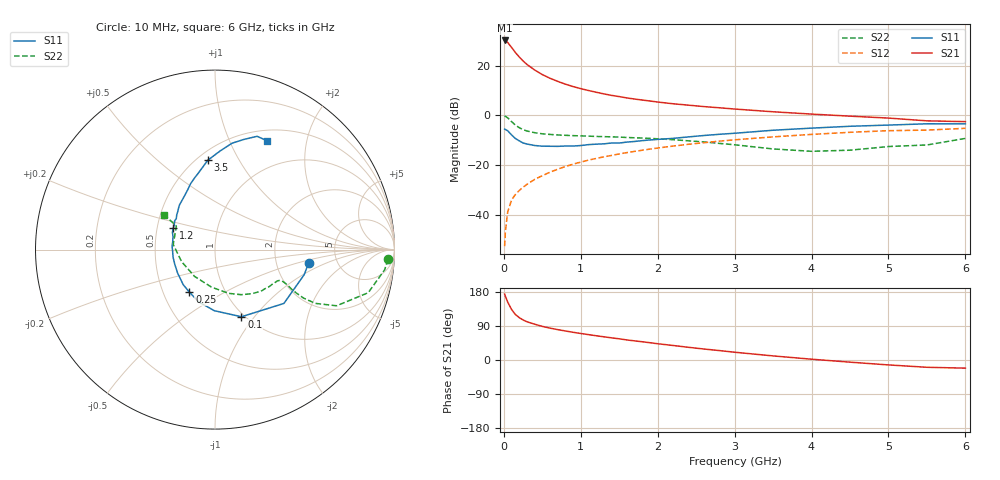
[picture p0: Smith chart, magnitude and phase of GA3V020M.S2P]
! Infineon Technologies  Discrete & RF Semiconductors
! BF775
! Si NPN RF Bipolar Junction Transistor in SOT23
! VCE = 3 V  IC = 20 mA
! Common Emitter S-Parameters:  May  1996
# GHz  S  MA  R  50
!  f  S11  S21  S12  S22
! GHz  MAG  ANG  MAG  ANG  MAG  ANG  MAG  ANG
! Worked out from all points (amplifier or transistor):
!   36 points, 10 MHz to 6 GHz, reference 50 ohm
!   highest |S21| = 30.2 dB at 10 MHz (marker M1)
!   |S21| within 3 dB of that: start of sweep to 105.4 MHz
!   unconditionally stable (mu >= 1): 387.8 MHz to 3.185 GHz
!   at 250 MHz: K = 0.88, MSG = 25.5 dB, |S12| = -29.0 dB
!   at 1.4 GHz: K = 1.12, MAG = 10.0 dB, |S12| = -16.2 dB
!   at 6 GHz: K = 0.96, MSG = 1.4 dB, |S12| = -5.3 dB
!   S11 on the Smith chart (normalised r, x): 10 MHz: 3.08, -0.63; 100 MHz: 0.97, -0.86; 250 MHz: 0.68, -0.35; 1.2 GHz: 0.61, +0.16; 3.5 GHz: 0.56, +0.75; 6 GHz: 0.63, +1.39
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0.01  0.5272 -8.1  32.22 174.0  0.0023 86.1  0.9659 -3.2
0.02  0.5162 -15.7  31.73 168.2  0.0045 84.6  0.9517 -6.8
0.05  0.4872 -38.0  29.27 152.8  0.0113 76.0  0.8871 -15.7
0.1  0.4021 -68.5  23.4 133.5  0.0196 68.2  0.7462 -24.8
0.15  0.3405 -90.6  18.45 120.1  0.0253 65.1  0.634 -28.2
0.2  0.3055 -107.1  14.97 111.9  0.0305 65.9  0.5626 -28.7
0.25  0.2767 -121.1  12.42 105.6  0.0354 66.7  0.5139 -28.1
0.3  0.2635 -132.3  10.6 100.9  0.0405 67.9  0.4826 -27.4
0.4  0.246 -147.9  8.199 94.5  0.051 68.8  0.4457 -25.9
0.5  0.2385 -160.3  6.607 88.7  0.0607 70.1  0.423 -25.3
0.6  0.2374 -169.6  5.573 84.1  0.0712 70.2  0.4107 -25.1
0.7  0.2363 -178.2  4.825 80.2  0.0819 70.0  0.4019 -25.4
0.8  0.24 175.3  4.237 76.6  0.0925 69.3  0.3948 -25.9
0.9  0.2397 169.4  3.795 73.1  0.1036 69.1  0.3888 -26.7
1.1  0.2561 158.0  3.158 67.0  0.1248 67.8  0.3798 -29.3
1.2  0.2617 152.8  2.914 64.0  0.135 66.9  0.3743 -30.5
1.6  0.2882 137.7  2.235 52.9  0.1769 62.9  0.3567 -37.0
2.2  0.3426 120.0  1.706 38.3  0.2393 56.2  0.3221 -49.5
3.5  0.4995 94.6  1.176 10.8  0.3671 39.4  0.2096 -95.6
4.5  0.6003 80.9  0.96 -5.7  0.4538 25.7  0.1978 -160.1
5.5  0.6735 69.6  0.772 -19.2  0.5027 10.8  0.2521 148.7
6  0.6723 64.3  0.745 -21.5  0.5459 6.5  0.342 145.5
